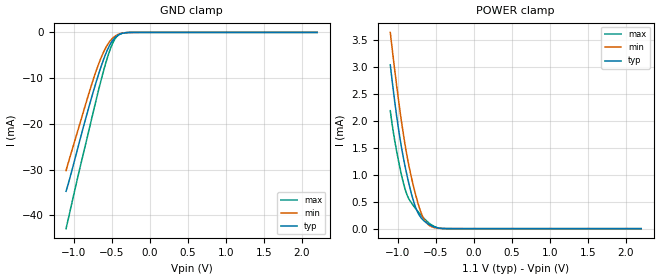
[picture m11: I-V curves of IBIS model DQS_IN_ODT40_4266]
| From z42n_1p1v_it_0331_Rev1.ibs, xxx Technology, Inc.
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| DQS_IN_ODT40_4266 (with 40ohm ODT, 3200-4266Mbps)
[Model]   DQS_IN_ODT40_4266
Model_type   Input
Vinl = 123.333mV
Vinh = 243.333mV
|   typ   min   max
|C_comp   0.809pF   0.766pF   0.862pF
C_comp_power_clamp   0.4045pF   0.3830pF   0.4310pF
C_comp_gnd_clamp   0.4045pF   0.3830pF   0.4310pF
| Note: C_comp changes when the ODT circuit is enabled.
[Model Spec]
| Input threshold voltage corners
Vinl   0.1233V   0.1167V   0.1350V
Vinh   0.2433V   0.2367V   0.2550V
| Dynamic Overshoot Parameters from LPDDR4 Specification
D_overshoot_ampl_h   0.30   NA   NA
D_overshoot_ampl_l   0.30   NA   NA
D_overshoot_area_h   0.1n   NA   NA
D_overshoot_area_l   0.1n   NA   NA
[Voltage Range]   1.1000V   1.0600V   1.1700V
[POWER Clamp Reference]   1.1000V   1.0600V   1.1700V
| Junction Temperature (Ambient temp is 35C typ 95C min -40C max)
[Temperature Range]   50.0   110.0   -40.0
[Add Submodel]
| Submodel Name   Mode
40ohm_ODT_4266   Non-Driving
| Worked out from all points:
|   GND clamp passes 1 mA (typ) near -0.45 V on its own axis
|   POWER clamp passes 1 mA (typ) near -0.88 V on its own axis
[GND Clamp]
|   Voltage   I(typ)   I(min)   I(max)
-1.1V     -34.74mA   -30.21mA   -42.91mA
-944.9mV  -25.23mA   -21.44mA   -31.56mA
-786.5mV  -15.53mA   -12.6mA    -20.49mA
-704mV    -10.84mA   -8.387mA   -14.74mA
-654.5mV  -8.229mA   -6.156mA   -11.42mA
-575.3mV  -4.574mA   -3.267mA   -6.539mA
-515.9mV  -2.484mA   -1.775mA   -3.512mA
-463.1mV  -1.249mA   -909.2uA   -1.597mA
-413.6mV  -575.8uA   -422.4uA   -623.6uA
-350.9mV  -168uA     -128.3uA   -147.4uA
-228.8mV  -7.219uA   -6.865uA   -4.033uA
2.2V      0A         0A         0A
[POWER Clamp]
|   Voltage   I(typ)   I(min)   I(max)
-1.1V     3.033mA    3.633mA    2.184mA
-1.041V   2.345mA    2.929mA    1.625mA
-981.2mV  1.753mA    2.275mA    1.183mA
-918.5mV  1.247mA    1.669mA    799.2uA
-855.8mV  837.7uA    1.173mA    553uA
-796.4mV  522uA      796.1uA    427.2uA
-743.6mV  316.1uA    512.4uA    330.1uA
-677.6mV  173uA      236.7uA    220.2uA
-601.7mV  87.05uA    76.12uA    117uA
-496.1mV  20.43uA    12.39uA    25.71uA
-387.2mV  1.97uA     1.327uA    1.64uA
2.2V      0A         0A         0A
